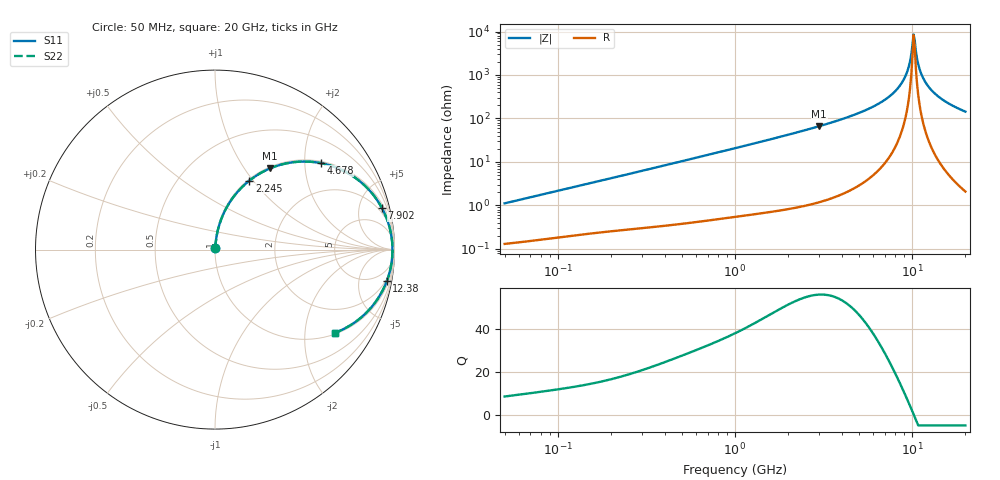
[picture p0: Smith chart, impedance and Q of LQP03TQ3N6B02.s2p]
!Murata Part Number: LQP03TQ3N6B02
!These Parameters are Measured in Series Mode Connection
!  o--[Z]--o
!Port1  Port2
!  o-------o
!Freq. Start=50[MHz] Stop=20[GHz], 401[Steps]
# Hz S RI R 50
!Freq.(Hz) S11(Real) S11(Imag) S21(Real) S21(Imag) S12(Real) S12(Imag) S22(Real) S22(Imag)
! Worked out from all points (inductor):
!   401 points, 50 MHz to 20 GHz, reference 50 ohm
!   read as one part in series: L = 3.49 nH near 51.52 MHz
!   highest Q = 56.1 at 2.985 GHz (marker M1), where L = 3.53 nH
!   self-resonance near 10.19 GHz
!   S11 on the Smith chart (normalised r, x): 50 MHz: 1.00, +0.02; 2.245 GHz: 1.02, +0.96; 4.678 GHz: 1.05, +2.40; 7.902 GHz: 1.39, +7.93; 12.38 GHz: 2, -11; 20 GHz: 1.04, -2.87
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5e7  0.00142 0.011  0.9986 -0.011  0.9986 -0.011  0.00142 0.011
1.364002e8  0.00297 0.029  0.997 -0.029  0.997 -0.029  0.00297 0.029
3.721004e8  0.00917 0.0764  0.9908 -0.0764  0.9908 -0.0764  0.00917 0.0764
1e9  0.0457 0.1962  0.9543 -0.1962  0.9543 -0.1962  0.0457 0.1962
2.245319e9  0.1914 0.3842  0.8086 -0.3842  0.8086 -0.3842  0.1914 0.3842
2.728004e9  0.2661 0.433  0.7339 -0.433  0.7339 -0.433  0.2661 0.433
2.98453e9  0.308 0.4528  0.692 -0.4528  0.692 -0.4528  0.308 0.4528
4.677679e9  0.5881 0.4821  0.4119 -0.4821  0.4119 -0.4821  0.5881 0.4821
6.125241e9  0.7831 0.3988  0.2169 -0.3988  0.2169 -0.3988  0.7831 0.3988
7.442007e9  0.902 0.2778  0.098 -0.2778  0.098 -0.2778  0.902 0.2778
7.901521e9  0.9304 0.2313  0.0696 -0.2313  0.0696 -0.2313  0.9304 0.2313
8.644534e9  0.9633 0.1551  0.0367 -0.1551  0.0367 -0.1551  0.9633 0.1551
9.178299e9  0.9781 0.1011  0.0219 -0.1011  0.0219 -0.1011  0.9781 0.1011
9.600142e9  0.9851 0.0595  0.0149 -0.0595  0.0149 -0.0595  0.9851 0.0595
1.004137e10  0.9885 0.0173  0.0115 -0.0173  0.0115 -0.0173  0.9885 0.0173
1.019291e10  0.9889 0.00313  0.0111 -0.00313  0.0111 -0.00313  0.9889 0.00313
1.050288e10  0.9883 -0.0251  0.0117 0.0251  0.0117 0.0251  0.9883 -0.0251
1.082228e10  0.9862 -0.0533  0.0138 0.0533  0.0138 0.0533  0.9862 -0.0533
1.115139e10  0.9824 -0.0813  0.0176 0.0813  0.0176 0.0813  0.9824 -0.0813
1.238412e10  0.957 -0.176  0.043 0.176  0.043 0.176  0.957 -0.176
1.504638e10  0.8659 -0.3273  0.1341 0.3273  0.1341 0.3273  0.8659 -0.3273
2e10  0.6707 -0.4628  0.3293 0.4628  0.3293 0.4628  0.6707 -0.4628
